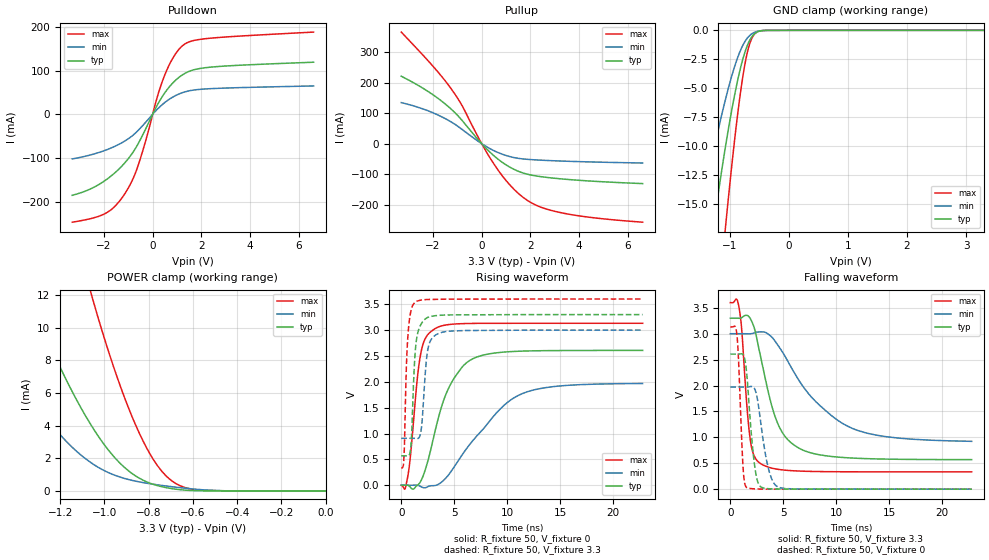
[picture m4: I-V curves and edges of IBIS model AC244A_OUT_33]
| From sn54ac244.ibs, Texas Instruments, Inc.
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[Model]   AC244A_OUT_33
Model_type  3-state
Enable   Active-Low
Vref =   0
Rref =   500
Cref =   50p
Vmeas =   1.65
| variable   typ   min   max
C_comp   5.14pF   4.71pF   5.55pF
| C_pullup   10.36pF   5.39pF   15.81pF
| C_pulldown   7.24pF   5.42pF   9.19pF
| C_tri-state   5.14pF   4.71pF   5.55pF
[Temperature Range]   40   100   -40
| Ambient temperature   25   85   -40
[Voltage range]   3.3   3   3.6
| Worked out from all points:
|   slope of the pulldown table from 0 to 0.495 V, typ, clamps not added: 10.1 ohm
|   slope of the pullup table from 0 to 0.495 V, typ, clamps not added: 12.7 ohm
|   GND clamp passes 1 mA (typ) near -0.68 V on its own axis
|   POWER clamp passes 1 mA (typ) near -0.87 V on its own axis
|   rising waveform, R_fixture 50, V_fixture 0: 20-80 % time 2.46ns typ, 4.74ns min, 909ps max; typ from 0 V to 2.61 V
|   falling waveform, R_fixture 50, V_fixture 3.3: 20-80 % time 2.2ns typ, 4.97ns min, 737ps max; typ from 3.3 V to 0.57 V
|   rising waveform, R_fixture 50, V_fixture 3.3: 20-80 % time 393ps typ, 475ps min, 323ps max; typ from 0.569 V to 3.3 V
|   falling waveform, R_fixture 50, V_fixture 0: 20-80 % time 643ps typ, 921ps min, 375ps max; typ from 2.61 V to 0 V
[GND Clamp]
| AC244A_OUT_33
|   Voltage   I(typ)   I(min)   I(max)
-3.3V     -118.7mA   -76.14mA   -162.3mA
-1.535V   -27.03mA   -16.93mA   -43.38mA
-1.295V   -17.52mA   -10.8mA    -29.01mA
-1.26V    -16.23mA   -9.974mA   -27mA
-1.085V   -10.28mA   -6.119mA   -17.41mA
-1.055V   -9.345mA   -5.516mA   -15.86mA
-925mV    -5.651mA   -3.167mA   -9.578mA
-790mV    -2.616mA   -1.362mA   -4.222mA
-700mV    -1.224mA   -624.9uA   -1.769mA
-600mV    -362.3uA   -206uA     -419.6uA
-385mV    -7.812uA   -5.806uA   -4.018uA
3.3V      17.55nA    87.16nA    85.27nA
[POWER Clamp]
| AC244A_OUT_33
|   Voltage   I(typ)   I(min)   I(max)
-3.3V     127.3mA    79.13mA    218.3mA
-1.615V   22.57mA    12.13mA    47.6mA
-1.365V   12.82mA    6.371mA    29.63mA
-1.325V   11.46mA    5.588mA    27.03mA
-1.085V   4.595mA    1.969mA    13.32mA
-1.05V    3.816mA    1.631mA    11.62mA
-945mV    1.919mA    921.8uA    7.072mA
-845mV    802.8uA    561.6uA    3.62mA
-780mV    407.2uA    411.9uA    1.951mA
-700mV    149.9uA    267uA      663.5uA
-550mV    5.986uA    64.1uA     29.92uA
0V        0A         0A         0A
[Pulldown]
| AC244A_OUT_33
|   Voltage   I(typ)   I(min)   I(max)
-3.3V     -185.8mA   -102.4mA   -247.4mA
-1.91V    -150.2mA   -81.88mA   -226.4mA
-1.505V   -131.9mA   -72.24mA   -208.3mA
-1.1V     -108.6mA   -59.82mA   -178.4mA
-810mV    -87.33mA   -48.18mA   -148.2mA
-580mV    -65.84mA   -36.08mA   -114.6mA
185mV     20.59mA    11.19mA    38.83mA
470mV     46.89mA    25.65mA    86.23mA
855mV     73.34mA    40.27mA    131.2mA
1.25V     91.25mA    49.99mA    158.3mA
2.385V    108mA      58.63mA    174.4mA
6.6V      119.2mA    64.84mA    188.3mA
[Pullup]
| AC244A_OUT_33
|   Voltage   I(typ)   I(min)   I(max)
-3.3V     220.7mA    134.4mA    365.1mA
-2.18V    169.7mA    106.9mA    269.6mA
-1.305V   116.7mA    73.55mA    185.3mA
-825mV    77.95mA    47.72mA    127.1mA
-30mV     2.661mA    1.591mA    4.365mA
500mV     -39.42mA   -22.81mA   -66.45mA
1.085V    -73.63mA   -40.72mA   -128.7mA
1.665V    -95.08mA   -49.69mA   -173.6mA
2.31V     -106.5mA   -53.47mA   -204.1mA
3.23V     -115mA     -56.72mA   -225.4mA
4.61V     -123mA     -60mA      -242.6mA
6.6V      -130.6mA   -63.26mA   -256.9mA
[Ramp]
| AC244A_OUT_33
| variable   typ   min   max
dV/dt_r   1.61/2.49E-09   1.21/4.81E-09   1.92/9.28E-10
dV/dt_f   1.67/2.21E-09   1.27/5.00E-09   2.00/7.51E-10
R_load = 50
[Rising Waveform]
| AC244A_OUT_33
R_fixture =   50
C_fixture =   0
L_fixture =   0
V_fixture =   0
V_fixture_min = 0
V_fixture_max = 0
|   Time   V(typ)   V(min)   V(max)
0s        132pV      309.2pV    44.78pV
355ps     397.1uV    -26.08uV   -70.85mV
675ps     -4.526mV   -49.96uV   242.7mV
1.525ns   504.3uV    -472.2uV   2.084V
1.88ns    92.39mV    -29.18mV   2.586V
3.205ns   1.057V     -5.093mV   3.03V
4.74ns    1.984V     277.8mV    3.112V
7.08ns    2.475V     940.6mV    3.13V
11.96ns   2.597V     1.812V     3.131V
22.79ns   2.607V     1.967V     3.131V
[Falling Waveform]
| AC244A_OUT_33
R_fixture =   50
C_fixture =   0
L_fixture =   0
V_fixture =   3.3
V_fixture_min = 3
V_fixture_max = 3.6
|   Time   V(typ)   V(min)   V(max)
0s        3.3V       3V         3.6V
815ps     3.298V     3V         3.516V
1.065ns   3.309V     3V         3.11V
1.555ns   3.355V     2.999V     1.633V
1.885ns   3.292V     2.999V     955.2mV
2.88ns    2.538V     3.036V     489.6mV
4.52ns    1.248V     2.771V     382.5mV
6.69ns    768.9mV    2.034V     348.1mV
12.1ns    594.9mV    1.128V     334.9mV
22.79ns   569.8mV    923mV      334mV
[Rising Waveform]
| AC244A_OUT_33
R_fixture =   50
C_fixture =   0
L_fixture =   0
V_fixture =   3.3
V_fixture_min = 3
V_fixture_max = 3.6
|   Time   V(typ)   V(min)   V(max)
0s        568.9mV    907.4mV    334mV
245ps     569.1mV    907.4mV    514.3mV
530ps     568.4mV    907.5mV    2.534V
870ps     681.1mV    907.8mV    3.328V
1.37ns    2.7V       904.9mV    3.547V
1.875ns   3.116V     1.064V     3.58V
2.315ns   3.223V     2.288V     3.59V
2.53ns    3.248V     2.646V     3.592V
3.42ns    3.283V     2.925V     3.595V
22.79ns   3.3V       3V         3.6V
[Falling Waveform]
| AC244A_OUT_33
R_fixture =   50
C_fixture =   0
L_fixture =   0
V_fixture =   0
V_fixture_min = 0
V_fixture_max = 0
|   Time   V(typ)   V(min)   V(max)
0s        2.607V     1.97V      3.131V
615ps     2.606V     1.971V     3.003V
765ps     2.607V     1.97V      2.543V
1.22ns    2.591V     1.97V      371.3mV
1.565ns   2.199V     1.971V     29.81mV
2.275ns   488.1mV    1.943V     5.717mV
2.925ns   39.12mV    1.204V     1.92mV
3.715ns   7.573mV    311.2mV    1.086mV
4.64ns    2.463mV    31.85mV    620.8uV
22.79ns   6.944uV    59.6uV     84.37nV
